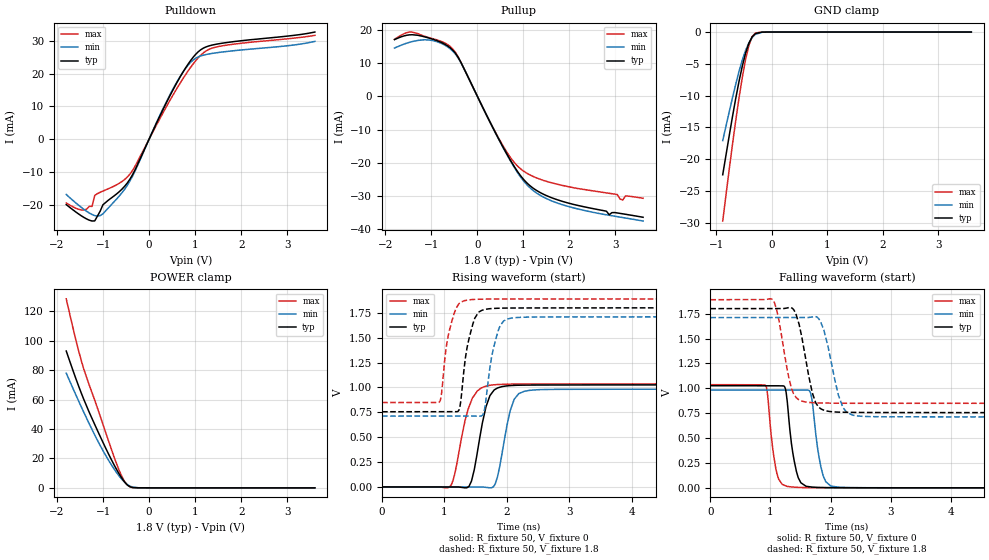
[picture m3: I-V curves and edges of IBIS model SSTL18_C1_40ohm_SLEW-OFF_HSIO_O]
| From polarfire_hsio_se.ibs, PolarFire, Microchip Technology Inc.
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|   Model SSTL18_C1_40ohm_SLEW-OFF_HSIO_O
[Model]   SSTL18_C1_40ohm_SLEW-OFF_HSIO_O
Model_type   Output
Polarity   Non-Inverting
Enable   Active-High
Vmeas =   0.9
Cref =   5p
Rref =   50
Vref =   0.9
|   typ   min   max
C_comp_pullup   1.335e-12   1.335e-12   1.380e-12
C_comp_pulldown  1.335e-12   1.335e-12   1.380e-12
[Temperature Range]  25C   100C   -40C
[Voltage Range]  1.8   1.71   1.89
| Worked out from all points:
|   slope of the pulldown table from 0 to 0.27 V, typ, clamps not added: 33.3 ohm
|   slope of the pullup table from 0 to 0.27 V, typ, clamps not added: 35.4 ohm
|   GND clamp passes 1 mA (typ) near -0.37 V on its own axis
|   POWER clamp passes 1 mA (typ) near -0.43 V on its own axis
|   rising waveform, R_fixture 50, V_fixture 0: 20-80 % time 187ps typ, 182ps min, 218ps max; typ from 0 V to 1.03 V
|   rising waveform, R_fixture 50, V_fixture 1.8: 20-80 % time 156ps typ, 162ps min, 153ps max; typ from 0.755 V to 1.8 V
|   falling waveform, R_fixture 50, V_fixture 0: 20-80 % time 131ps typ, 134ps min, 116ps max; typ from 1.03 V to 0 V
|   falling waveform, R_fixture 50, V_fixture 1.8: 20-80 % time 198ps typ, 222ps min, 185ps max; typ from 1.8 V to 0.755 V
[GND Clamp]
| Voltage   I(typ)   I(min)   I(max)
-885.9mV  -22.44mA   -17.06mA   -29.71mA
-708.7mV  -13.24mA   -10.28mA   -17.6mA
-649.7mV  -10.37mA   -8.138mA   -13.83mA
-590.6mV  -7.705mA   -6.148mA   -10.3mA
-531.6mV  -5.322mA   -4.371mA   -7.074mA
-472.5mV  -3.308mA   -2.865mA   -4.286mA
-413.4mV  -1.757mA   -1.684mA   -2.101mA
-354.4mV  -739.5uA   -855.1uA   -713.7uA
-295.3mV  -232.3uA   -363.2uA   -148.3uA
-177.2mV  -12.01uA   -39.02uA   -3.177uA
-59.06mV  -489.8nA   -2.616uA   -234.3nA
3.6V      0A         0A         0A
[POWER Clamp]
| Voltage   I(typ)   I(min)   I(max)
-1.8V     93.11mA    78.02mA    128.6mA
-1.595V   74.64mA    63.48mA    101.1mA
-1.477V   64.73mA    55.33mA    86.9mA
-1.417V   60.07mA    51.32mA    80.62mA
-1.063V   35.01mA    28.82mA    48.84mA
-885.9mV  23.32mA    19.01mA    32.31mA
-708.7mV  12.62mA    10.48mA    16.53mA
-590.6mV  6.476mA    5.751mA    7.626mA
-472.5mV  1.932mA    2.149mA    1.873mA
-354.4mV  154uA      469.9uA    209.6uA
-236.2mV  4.969uA    79.11uA    56.46uA
3.6V      0A         0A         0A
[Pullup]
| Voltage   I(typ)   I(min)   I(max)
-1.8V     17.05mA    14.51mA    17.13mA
-1.417V   18.52mA    16.45mA    19.33mA
-945mV    17.06mA    16.68mA    17.24mA
-531.6mV  13.85mA    13.56mA    14.2mA
-354.4mV  10.14mA    10.03mA    10.16mA
618.8mV   -16.82mA   -16.96mA   -16.3mA
900mV     -23.17mA   -23.51mA   -21.35mA
1.238V    -27.89mA   -28.62mA   -24.28mA
1.859V    -31.66mA   -32.67mA   -26.85mA
2.863V    -35.64mA   -35.8mA    -29.19mA
3.158V    -35.36mA   -36.49mA   -31.2mA
3.6V      -36.4mA    -37.52mA   -30.68mA
[Pulldown]
| Voltage   I(typ)   I(min)   I(max)
-1.8V     -19.98mA   -16.9mA    -19.49mA
-1.477V   -23.37mA   -20.8mA    -21.61mA
-1.24V    -25mA      -23.01mA   -20.53mA
-1.181V   -24.96mA   -23.35mA   -17.16mA
-1.004V   -20.05mA   -22.8mA    -15.86mA
-649.7mV  -16.06mA   -17.4mA    -13.5mA
-413.4mV  -12.15mA   -12.7mA    -10.62mA
562.5mV   16.17mA    16.44mA    14.49mA
843.8mV   22.82mA    22.52mA    20.76mA
1.125V    27.3mA     25.4mA     25.66mA
1.575V    29.24mA    26.55mA    28.43mA
3.6V      32.67mA    29.82mA    31.66mA
[Ramp]
dV/dt_r   0.61537/0.186847n  0.589455/0.181546n  0.621704/0.218129n
dV/dt_f   0.62673/0.197632n  0.598698/0.222311n  0.625121/0.184841n
R_load = 50
[Rising Waveform]
R_fixture = 50
V_fixture = 0
V_fixture_min = 0
V_fixture_max = 0
| Time   V(typ)   V(min)   V(max)
0s        2.38uV     2.517uV    4.62uV
1.096ns   -743.4uV   -579.1uV   9.113mV
1.393ns   5.215mV    -736.7uV   803.6mV
1.527ns   348.5mV    -807.8uV   964.9mV
1.723ns   907.5mV    -8.653mV   1.021V
1.849ns   994mV      99.14mV    1.029V
2.003ns   1.016V     623.6mV    1.033V
2.118ns   1.02V      881.6mV    1.034V
2.283ns   1.023V     961.9mV    1.034V
10ns      1.026V     982.4mV    1.036V
[Rising Waveform]
R_fixture = 50
V_fixture = 1.8
V_fixture_min = 1.71
V_fixture_max = 1.89
| Time   V(typ)   V(min)   V(max)
0s        755.4mV    712.1mV    848.1mV
919ps     756.1mV    712.2mV    853.4mV
1.061ns   756.2mV    712.2mV    1.521V
1.233ns   774.1mV    712.2mV    1.842V
1.375ns   1.437V     712.2mV    1.879V
1.486ns   1.696V     712.2mV    1.884V
1.618ns   1.778V     728.4mV    1.887V
1.861ns   1.796V     1.569V     1.888V
2.082ns   1.798V     1.697V     1.889V
10ns      1.8V       1.71V      1.89V
[Falling Waveform]
R_fixture = 50
V_fixture = 0
V_fixture_min = 0
V_fixture_max = 0
| Time   V(typ)   V(min)   V(max)
0s        1.026V     982.4mV    1.036V
919ps     1.025V     981.9mV    1.028V
1.105ns   1.025V     981.8mV    146.7mV
1.277ns   873.2mV    981.7mV    14.65mV
1.348ns   444mV      981.7mV    8.684mV
1.461ns   101.5mV    981.6mV    4.592mV
1.668ns   9.549mV    948.4mV    2.14mV
1.835ns   3.633mV    216.2mV    1.487mV
1.999ns   2.054mV    19.47mV    1.143mV
10ns      3.459uV    3.354uV    5.045uV
[Falling Waveform]
R_fixture = 50
V_fixture = 1.8
V_fixture_min = 1.71
V_fixture_max = 1.89
| Time   V(typ)   V(min)   V(max)
0s        1.8V       1.71V      1.89V
1.026ns   1.801V     1.711V     1.894V
1.099ns   1.801V     1.711V     1.797V
1.386ns   1.789V     1.711V     942.3mV
1.585ns   1.294V     1.711V     862.4mV
1.695ns   953mV      1.717V     855.5mV
1.798ns   812.3mV    1.701V     853mV
2.128ns   760.6mV    931.3mV    850mV
2.372ns   758mV      728.9mV    849.3mV
10ns      755.4mV    712.1mV    848.1mV
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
